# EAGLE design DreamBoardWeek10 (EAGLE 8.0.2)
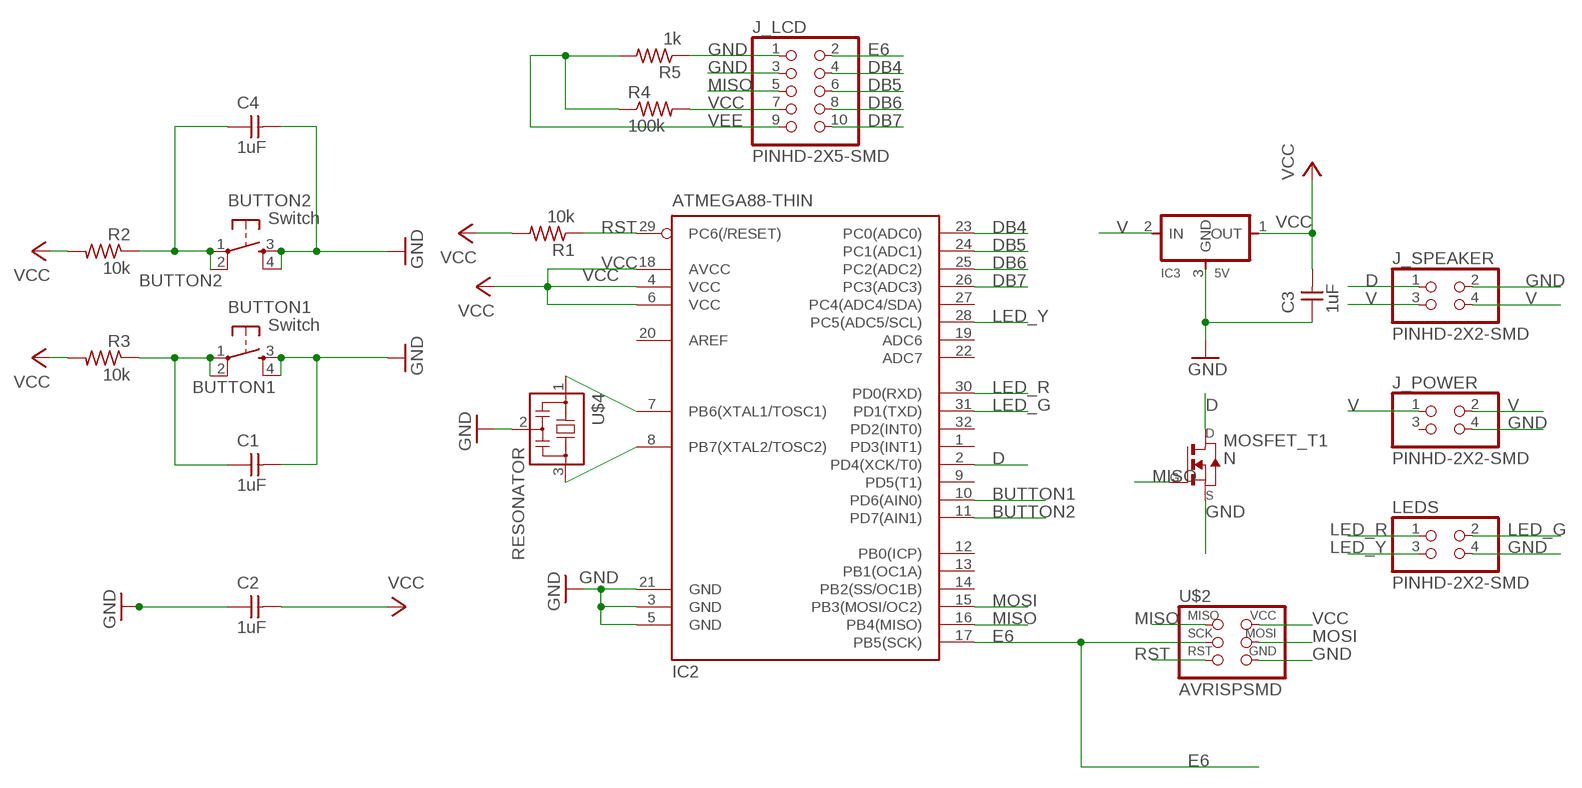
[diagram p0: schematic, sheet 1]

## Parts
BUTTON1  Switch  6MM_SWITCH6MM_SWITCH  [6MM_SWITCH]
BUTTON2  Switch  6MM_SWITCH6MM_SWITCH  [6MM_SWITCH]
C1  1uF  CAP-UNPOLARIZEDFAB  [C1206FAB]
C2  1uF  CAP-UNPOLARIZEDFAB  [C1206FAB]
C3  1uF  CAP-UNPOLARIZEDFAB  [C1206FAB]
C4  1uF  CAP-UNPOLARIZEDFAB  [C1206FAB]
IC2  ATMEGA88-THIN  [TQFP32-08THIN]
IC3  5V  REGULATORSOT23  [SOT23]
J_LCD  PINHD-2X5-SMD  [2X05SMD]
J_POWER  PINHD-2X2-SMD  [2X02SMD]
J_SPEAKER  PINHD-2X2-SMD  [2X02SMD]
LEDS  PINHD-2X2-SMD  [2X02SMD]
MOSFET_T1  N  NMOSFETSOT23  [SOT-23]
R1  10k  RES-US1206FAB  [R1206FAB]
R2  10k  RES-US1206FAB  [R1206FAB]
R3  10k  RES-US1206FAB  [R1206FAB]
R4  100k  RES-US1206FAB  [R1206FAB]
R5  1k  RES-US1206FAB  [R1206FAB]
U$2  AVRISPSMD  [2X03SMD]
U$4  RESONATOR  [EFOBM]

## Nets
BUTTON1: BUTTON1.1(P) BUTTON1.2(P1) C1.1 IC2.10(PD6(AIN0)) R3.1
BUTTON2: BUTTON2.1(P) BUTTON2.2(P1) C4.1 IC2.11(PD7(AIN1)) R2.1
D: IC2.2(PD4(XCK/T0)) J_SPEAKER.1 MOSFET_T1.1(D)
DB4: IC2.23(PC0(ADC0)) J_LCD.4
DB5: IC2.24(PC1(ADC1)) J_LCD.6
DB6: IC2.25(PC2(ADC2)) J_LCD.8
DB7: IC2.26(PC3(ADC3)) J_LCD.10
E6: IC2.17(PB5(SCK)) J_LCD.2 U$2.3(SCK)
GND: BUTTON1.3(S) BUTTON1.4(S1) BUTTON2.3(S) BUTTON2.4(S1) C1.2 C2.1 C3.1 C4.2 IC2.3(GND) IC2.5(GND) IC2.21(GND) IC3.3(GND) J_LCD.1 J_LCD.3 J_POWER.4 J_SPEAKER.2 LEDS.4 MOSFET_T1.2(S) R5.1 U$2.6(GND) U$4.2
LED_G: IC2.31(PD1(TXD)) LEDS.2
LED_R: IC2.30(PD0(RXD)) LEDS.1
LED_Y: IC2.28(PC5(ADC5/SCL)) LEDS.3
MISO: IC2.16(PB4(MISO)) J_LCD.5 MOSFET_T1.3(G) U$2.1(MISO)
MOSI: IC2.15(PB3(MOSI/OC2)) U$2.4(MOSI)
N$1: IC2.8(PB7(XTAL2/TOSC2)) U$4.3
N$2: IC2.7(PB6(XTAL1/TOSC1)) U$4.1
RST: IC2.29(PC6(/RESET)) R1.1 U$2.5(RST)
V: IC3.2(IN) J_POWER.1 J_POWER.2 J_SPEAKER.3 J_SPEAKER.4
VCC: C2.2 C3.2 IC2.4(VCC) IC2.6(VCC) IC2.18(AVCC) IC3.1(OUT) J_LCD.7 R1.2 R2.2 R3.2 R4.2 U$2.2(VCC)
VEE: J_LCD.9 R4.1 R5.2
Unconnected: IC2.1(PD3(INT1)) IC2.9(PD5(T1)) IC2.12(PB0(ICP)) IC2.13(PB1(OC1A)) IC2.14(PB2(SS/OC1B)) IC2.19(ADC6) IC2.20(AREF) IC2.22(ADC7) IC2.27(PC4(ADC4/SDA)) IC2.32(PD2(INT0)) J_POWER.3

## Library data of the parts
BUTTON1 BUTTON2 = fab:6MM_SWITCH: OMRON SWITCH
C1-C4 = fab:CAP-UNPOLARIZED
IC2 = fab:ATMEGA88-THIN
IC3 = fab:REGULATOR
J_LCD = fab:PINHD-2X5-SMD
J_POWER J_SPEAKER LEDS = fab:PINHD-2X2-SMD
MOSFET_T1 = fab:NMOSFET: MOS FET
R1-R5 = fab:RES-US: Resistor (US Symbol)
U$2 = fab:AVRISP
U$4 = fab:RESONATOR

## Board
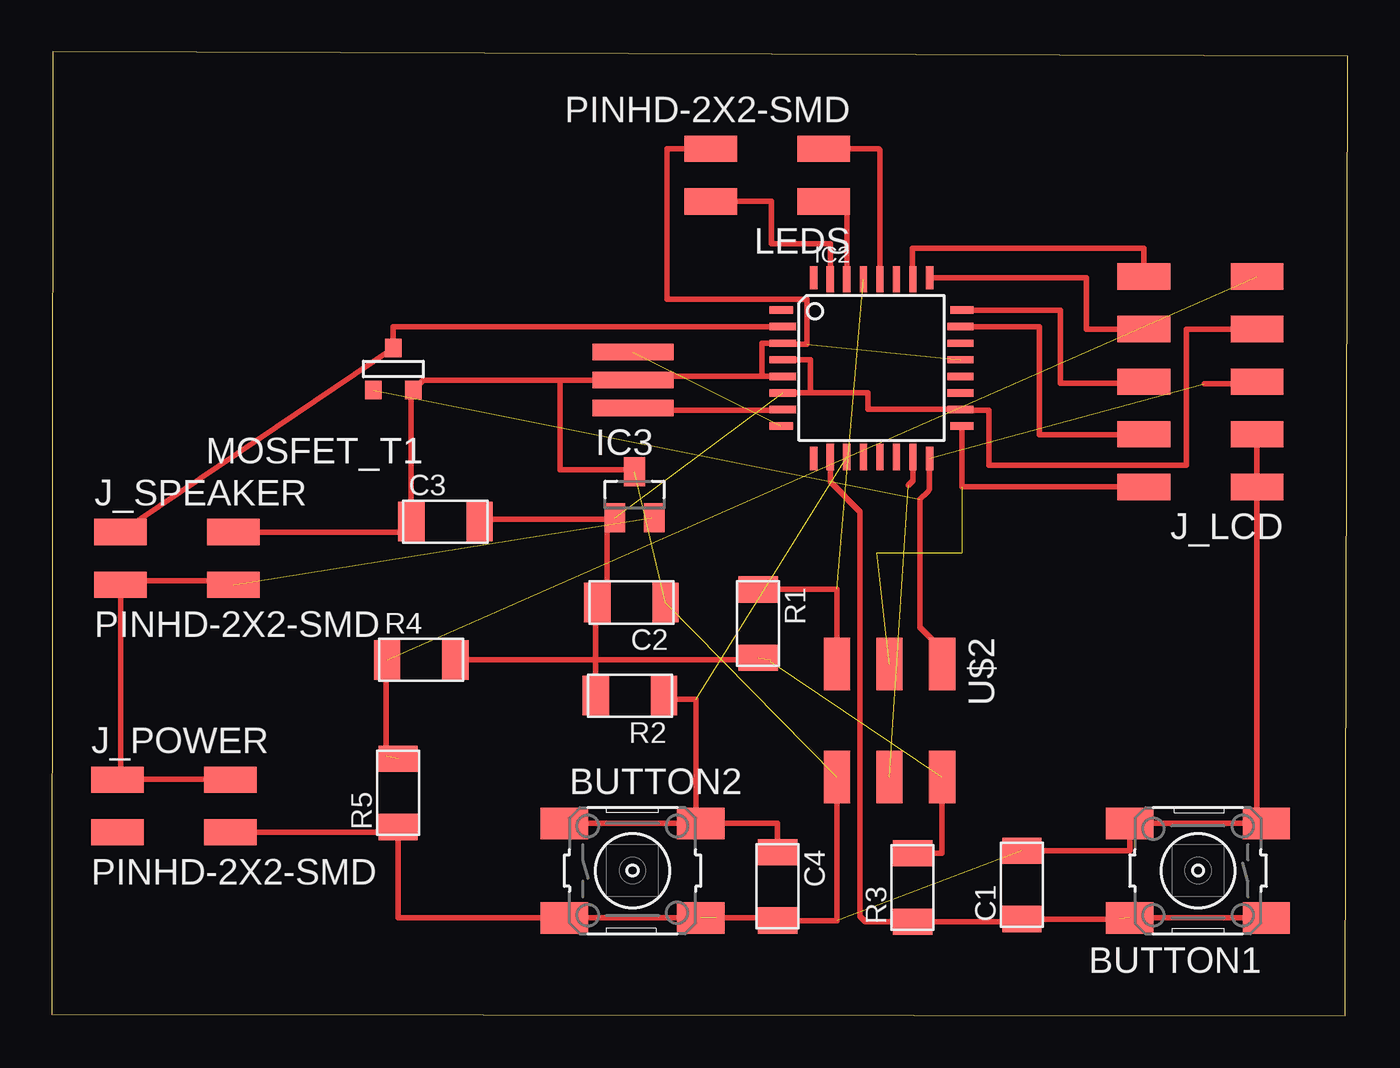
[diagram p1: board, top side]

Size 62.64 x 46.57 mm. Coordinates in mm from the lower left corner, seen from the top.
Outline: 0,0.08 62.51,0 62.64,46.35 0.05,46.57 0,0.08
Copper layers (1*16): Top 0.035mm / dielectric 1.5mm / Bottom 0.035mm
Design rules "default *": minimum track width 10mil, minimum drill 24mil, track to track 16mil, track to pad 16mil, pad to pad 16mil, via to via 16mil, smd to smd 8mil, copper to edge 40mil, drill to drill 8mil, minimum pad ring 10mil, minimum via ring 8mil, stop-mask expansion 4mil, vias tented up to drill 0mil, thermal gap 10mil

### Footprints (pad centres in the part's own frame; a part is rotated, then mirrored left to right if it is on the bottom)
6MM_SWITCH = smd 2.286 x 1.524: 1 -3.302,2.286; 2 3.302,2.286; 3 -3.302,-2.286; 4 3.302,-2.286
C1206FAB = smd 1.27 x 1.905: 1 -1.651,0; 2 1.651,0
TQFP32-08THIN = smd 1.118 x 0.356: 1 -4.369,2.8; 8 -4.369,-2.8; 17 4.369,-2.8; 24 4.369,2.8 | smd 1.27 x 0.356: 2 -4.293,2; 3 -4.293,1.2; 4 -4.293,0.4; 5 -4.293,-0.4; 6 -4.293,-1.2; 7 -4.293,-2; 18 4.293,-2; 19 4.293,-1.2; 20 4.293,-0.4; 21 4.293,0.4; 22 4.293,1.2; 23 4.293,2 | smd 0.356 x 1.118: 9 -2.8,-4.369; 16 2.8,-4.369; 25 2.8,4.369; 32 -2.8,4.369 | smd 0.356 x 1.27: 10 -2,-4.293; 14 1.2,-4.293; 15 2,-4.293; 26 2,4.293; 27 1.2,4.293; 31 -2,4.293 | smd 0.35 x 1.27: 11 -1.2,-4.293; 12 -0.4,-4.293; 13 0.4,-4.293; 28 0.4,4.293; 29 -0.4,4.293; 30 -1.2,4.293
SOT23 = smd 1 x 1.4: 1 -0.95,-1.1; 2 0.95,-1.1; 3 0,1.1
2X05SMD = smd 2.54 x 1.27: 1 -2.54,2.54; 2 2.92,2.54; 3 -2.54,0; 4 2.92,0; 5 -2.54,-2.54; 6 2.92,-2.54; 7 -2.54,-5.08; 8 2.92,-5.08; 9 -2.54,-7.62; 10 2.92,-7.62
2X02SMD = smd 2.54 x 1.27: 1 -2.54,1.27; 2 2.92,1.27; 3 -2.54,-1.27; 4 2.92,-1.27
SOT-23 = smd 0.787 x 0.889: 1 0.025,-1.016; 2 -0.94,1.016; 3 0.991,1.016
R1206FAB = smd 1.27 x 1.905: 1 -1.651,0; 2 1.651,0
2X03SMD = smd 2.54 x 1.27: 1 -2.54,2.54; 2 2.92,2.54; 3 -2.54,0; 4 2.92,0; 5 -2.54,-2.54; 6 2.92,-2.54
EFOBM = smd 0.8 x 3.9: 1 -1.35,0; 2 0,0; 3 1.35,0

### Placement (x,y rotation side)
BUTTON1  55.4,7.01 180 top
BUTTON2  28.07,7.01 0 top
C1  46.89,6.32 90 top
C2  28.02,19.96 180 top
C3  19.02,23.88 0 top
C4  35.08,6.25 270 top
IC2  39.62,31.29 0 top
IC3  28.17,25.17 0 top
J_LCD  55.7,28.09 180 top
J_POWER  5.71,10.13 0 top
J_SPEAKER  5.87,22.1 0 top
LEDS  34.77,40.61 180 top
MOSFET_T1  16.54,31.24 180 top
R1  34.14,18.95 270 top
R2  27.94,15.47 180 top
R3  41.61,6.2 90 top
R4  17.86,17.2 0 top
R5  16.74,10.77 90 top
U$2  40.49,14.45 270 top
U$4  28.09,30.71 90 top

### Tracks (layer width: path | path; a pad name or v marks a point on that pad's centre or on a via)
BUTTON1  (1 unrouted)
  Top 0.254: 51.59,4.7 51.59,4.52 | BUTTON1.1 BUTTON1.2 52.1,4.67 C1.1 46.89,4.55 R3.1 39.32,4.55 39.07,4.8 39.07,24.36 37.62,25.8 IC2.10
BUTTON2  (1 unrouted)
  Top 0.254: 29.41,15.39 R2.1 29.59,15.29 31.14,15.29 31.14,9.3 BUTTON2.2 | BUTTON2.2 BUTTON2.1 | C4.1 35.08,9.3 BUTTON2.2
D
  Top 0.254: J_SPEAKER.1 MOSFET_T1.1 16.51,33.29 IC2.2
DB4
  Top 0.254: IC2.23 47.73,33.29 47.73,28.07 52.78,28.07 J_LCD.4
DB5
  Top 0.254: IC2.24 48.74,34.09 48.74,30.56 52.78,30.56 J_LCD.6
DB6
  Top 0.254: IC2.25 50.01,35.66 50.01,33.17 J_LCD.8
DB7
  Top 0.254: IC2.26 41.61,35.59 41.61,37.08 52.78,37.08 J_LCD.10
E6  (3 unrouted)
  Top 0.254: IC2.17 43.99,25.55 J_LCD.2
GND  (5 unrouted)
  Top 0.254: 28.09,26.29 IC3.3 28.17,26.39 24.56,26.39 24.56,30.71 U$4.2 | 58.47,9.45 BUTTON1.3 arc-90 58.24,9.75 | 52.2,9.45 BUTTON1.4 | 8.94,9.12 J_POWER.4 16.74,8.86 R5.1 16.74,4.72 BUTTON2.3 32.11,4.72 32.11,4.34 | C3.1 17.3,23.88 17.3,24.38 | C3.1 17.37,30.23 MOSFET_T1.2 17.96,30.71 U$4.2 | J_SPEAKER.2 17.37,23.37 C3.1 | U$4.2 29.67,30.71 29.67,30.94 29.9,30.94 29.9,30.89 34.32,30.89 | 34.32,30.89 IC2.5 | 58.65,28.09 J_LCD.3 J_LCD.1 58.24,9.75 | BUTTON1.4 51.94,9.3 | 34.32,30.89 34.32,32.49 IC2.3 35.33,32.44 36.5,32.44 36.5,34.62 29.74,34.62 29.74,41.88 LEDS.4 | BUTTON2.4 34.95,4.72 C4.2 | C4.2 35.08,4.62 | C4.2 35.08,4.57 | C1.2 52.1,7.98 BUTTON1.4 | BUTTON1.4 58.24,9.3 58.24,9.75 | C4.2 37.95,4.6 U$2.6
LED_G
  Top 0.254: LEDS.2 34.77,39.34 34.77,37.29 37.62,37.29 IC2.31
LED_R
  Top 0.254: LEDS.1 38.42,39.32 IC2.30
LED_Y
  Top 0.254: 37.08,41.88 LEDS.3 39.95,41.88 40.02,41.81 IC2.28
MISO  (2 unrouted)
  Top 0.254: 55.7,30.53 58.24,30.53 J_LCD.5 | IC2.16 42.42,25.43 42.34,25.32 41.96,24.94 41.96,18.77 43.03,17.7 U$2.1
MOSI  (1 unrouted)
  Top 0.254: 41.63,26.95 IC2.15 | IC2.15 41.58,27 | 41.4,25.63 41.63,25.86 41.63,26.82 IC2.15
N$1  (1 unrouted)
N$2
  Top 0.254: IC2.7 35.03,29.26 28.09,29.26 U$4.1
RST  (1 unrouted)
  Top 0.254: 37.85,16.99 U$2.5 37.95,20.6 R1.1
V  (1 unrouted)
  Top 0.254: 3.33,11.43 8.61,11.43 J_POWER.2 | J_SPEAKER.4 8.61,21.01 3.33,21.01 J_SPEAKER.3 3.33,11.43 | 3.33,11.43 J_POWER.1 | IC3.2 28.98,24.07
VCC  (3 unrouted)
  Top 0.254: C2.2 26.11,19.69 | C3.2 20.83,23.98 27.1,23.98 IC3.1 26.85,24.07 26.85,20.27 26.37,20.27 C2.2 | 26.44,15.39 R2.2 26.29,17.2 | 26.37,19.81 C2.2 | C2.2 26.29,19.96 26.29,17.2 | J_LCD.7 54.84,33.17 54.84,26.59 45.29,26.59 45.29,29.26 43.92,29.26 IC2.18 43.92,29.31 39.45,29.31 39.45,30.09 36.68,30.09 | R4.2 26.29,17.2 | 36.68,30.09 IC2.6 | IC2.4 36.68,31.69 36.68,30.09 | R3.2 43.03,7.85 U$2.2 43.03,11.46 | 26.29,17.2 34.75,17.2 34.75,17.09
VEE  (2 unrouted)
  Top 0.254: R4.1 16.15,17.2 16.15,12.55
